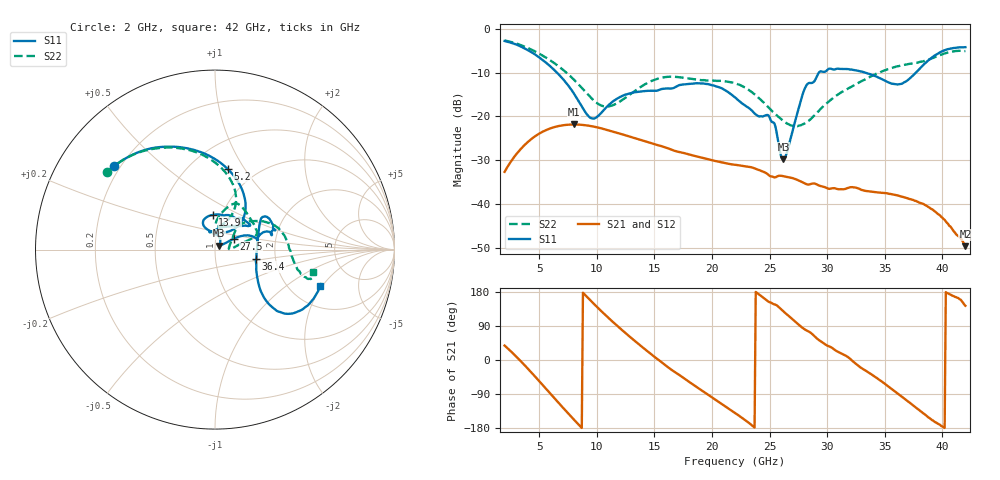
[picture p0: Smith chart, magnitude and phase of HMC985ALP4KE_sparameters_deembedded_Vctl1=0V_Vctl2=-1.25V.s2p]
!s2p File: Measurements: S11, S21, S12, S22
# GHz S dB R 50.0
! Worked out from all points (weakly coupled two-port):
!   401 points, 2 GHz to 42 GHz, reference 50 ohm
!   highest |S21| = -21.82 dB at 8 GHz (marker M1); lowest = -49.7 dB at 42 GHz (marker M2)
!   lowest |S11| = -29.8 dB at 26.2 GHz (marker M3), VSWR 1.07, Z = 52.4 + j2.28 ohm
!   |S11| at or under -10 dB: 6.559 GHz to 29.27 GHz (22.71 GHz wide, 127 % of centre); 33.35 GHz to 37.69 GHz (4.344 GHz wide, 12.2 % of centre)
!   |S22| runs from -22.2 to -2.6 dB; largest |S21 - S12| = 0.00017
!   S11 on the Smith chart (normalised r, x): 2 GHz: 0.18, +0.35; 5.2 GHz: 0.75, +0.84; 13.9 GHz: 0.90, +0.36; 27.5 GHz: 1.22, +0.15; 36.4 GHz: 1.58, -0.18; 42 GHz: 2.90, -1.91
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2  -2.73 140.5  -32.67 38.1  -32.69 38.1  -2.61 144.1
3.5  -4.12 112.8  -27.16 -6.2  -27.16 -6.1  -3.77 119.3
5.2  -6.87 80.8  -23.63 -62.4  -23.63 -62.4  -5.92 93.3
8  -14.68 45.9  -21.82 -156.8  -21.83 -156.8  -11.53 64.9
8.7  -17.73 51.9  -21.91 -179.3  -21.91 -179.3  -13.47 64.3
9.7  -20.48 85.1  -22.29 149.6  -22.29 149.6  -16.25 70.7
10.9  -17.71 113.4  -23.07 114.4  -23.07 114.3  -17.72 84.5
13.9  -14.25 93.9  -25.43 35.4  -25.43 35.4  -13.09 77.5
15.4  -13.94 73.0  -26.64 -0.5  -26.65 -0.5  -11.28 68.5
19.4  -12.52 34.5  -29.63 -86.2  -29.64 -86.3  -11.72 36.9
22  -15.62 52.3  -31.04 -139.6  -31.05 -139.6  -12.40 18.8
25  -20.17 98.0  -33.57 152.5  -33.56 152.5  -18.18 9.8
26.2  -29.79 42.2  -33.66 128.4  -33.66 128.3  -21.03 2.6
27.5  -18.39 29.8  -34.62 93.7  -34.63 93.6  -22.13 6.4
28.1  -13.35 20.8  -35.36 79.9  -35.36 79.8  -21.53 15.2
28.7  -12.31 12.9  -35.35 68.5  -35.38 68.6  -20.26 24.6
31  -9.08 23.4  -36.65 20.7  -36.62 20.7  -14.85 45.0
33.3  -9.96 34.4  -37.01 -27.2  -37.00 -27.2  -11.52 36.6
35.4  -12.27 12.3  -37.70 -71.8  -37.71 -71.8  -9.09 23.2
36.4  -12.57 -12.9  -38.28 -95.0  -38.27 -95.1  -8.31 15.6
39.5  -5.80 -43.3  -42.03 -165.8  -42.05 -166.6  -6.25 -14.4
42  -4.14 -19.0  -49.66 143.2  -49.71 142.5  -5.04 -13.0
